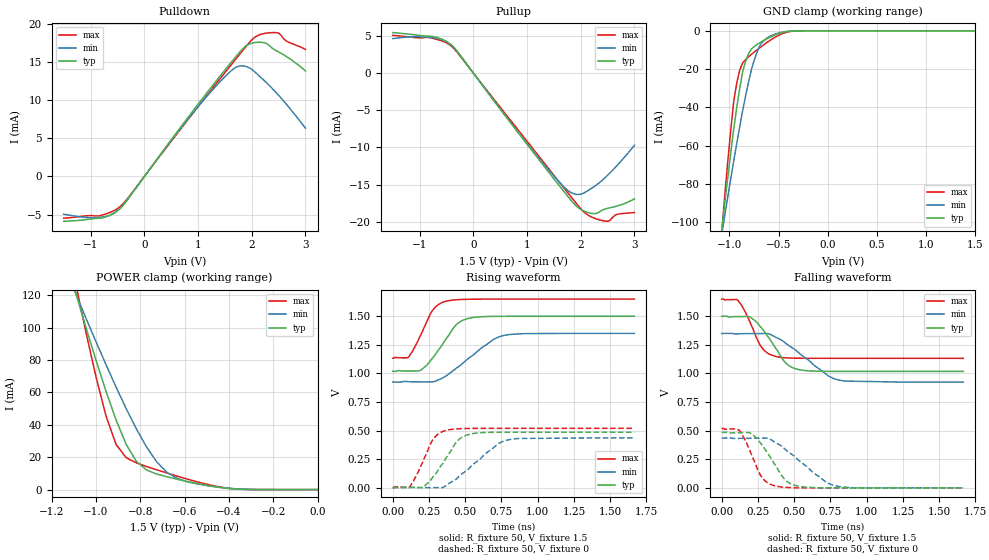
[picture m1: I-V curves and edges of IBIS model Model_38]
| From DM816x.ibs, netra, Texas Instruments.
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| Model based on original model for BSHTLTCSCDVGPBFZ
|   Sub model SLOWEST_4MA_10PER_1P5
[model]   Model_38
|[Description]  1.5V-3-STATE-X-SLOWEST, 4MA, +-10%
|[Input Load]
|[Output Drive] SLOWEST, 4MA
|Voltage   1.5V
|Mode   3-STATE
Model_type   3-state
Polarity   Non-Inverting
Enable   Active-Low
Cref =  15.0000pF
Rref =  100.0000M
Vref =  0V
Vmeas =  0.75
C_comp   1.5249p   1.4275p   1.6205p
[Model Spec]
[Temperature Range]   25   125   -40
[Voltage Range]   1.5   1.35   1.65
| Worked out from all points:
|   slope of the pulldown table from 0 to 0.225 V, typ, clamps not added: 103 ohm
|   slope of the pullup table from 0 to 0.225 V, typ, clamps not added: 103 ohm
|   GND clamp passes 1 mA (typ) near -0.47 V on its own axis
|   POWER clamp passes 1 mA (typ) near -0.42 V on its own axis
|   rising waveform, R_fixture 50, V_fixture 1.5: 20-80 % time 161ps typ, 258ps min, 118ps max; typ from 1.02 V to 1.5 V
|   rising waveform, R_fixture 50, V_fixture 0: 20-80 % time 154ps typ, 247ps min, 114ps max; typ from 0 V to 0.485 V
|   falling waveform, R_fixture 50, V_fixture 1.5: 20-80 % time 155ps typ, 264ps min, 113ps max; typ from 1.5 V to 1.02 V
|   falling waveform, R_fixture 50, V_fixture 0: 20-80 % time 150ps typ, 254ps min, 109ps max; typ from 0.485 V to 0 V
[POWER_clamp]
-1.5V     321.6mA    260.6mA    415.8mA
-1.091V   121.1mA    120.8mA    126.6mA
-1.076V   114.1mA    115.8mA    116.8mA
-1V       79.88mA    91.3mA     69.56mA
-954.5mV  60.58mA    77.05mA    45.34mA
-909.1mV  42.84mA    63.2mA     27.8mA
-818.2mV  17.47mA    37.6mA     16.51mA
-772.7mV  12.19mA    26.53mA    14.33mA
-681.8mV  7.985mA    10.89mA    10.33mA
-590.9mV  5.092mA    4.952mA    6.596mA
-363.6mV  298.9uA    465.6uA    298.1uA
0V        1.518nA    23.05nA    396.5pA
[Pulldown]
-1.5V     -5.88mA    -4.94mA    -5.47mA
-863.6mV  -5.487mA   -5.379mA   -5.186mA
-500mV    -4.486mA   -4.503mA   -4.211mA
-318.2mV  -3.077mA   -3.07mA    -2.94mA
1V        9.473mA    9.16mA     9.156mA
1.455V    13.57mA    12.77mA    13.23mA
1.727V    15.92mA    14.4mA     15.62mA
1.955V    17.38mA    14.26mA    17.57mA
2.273V    17.45mA    12.32mA    18.81mA
2.5V      16.34mA    10.65mA    18.81mA
2.636V    15.78mA    9.54mA     17.81mA
3V        13.85mA    6.33mA     16.67mA
[Pullup]
-1.5V     5.43mA     4.62mA     5.06mA
-772.7mV  4.923mA    4.757mA    4.681mA
-409.1mV  3.79mA     3.753mA    3.62mA
1.227V    -11.69mA   -11.51mA   -11.25mA
1.682V    -15.87mA   -15.27mA   -15.39mA
1.864V    -17.48mA   -16.22mA   -17.03mA
2V        -18.33mA   -16.3mA    -18.23mA
2.182V    -18.84mA   -15.6mA    -19.29mA
2.409V    -18.4mA    -14.37mA   -19.84mA
2.545V    -18.12mA   -13.43mA   -19.81mA
2.682V    -17.87mA   -12.4mA    -18.99mA
3V        -16.92mA   -9.72mA    -18.75mA
[GND_clamp]
-1.5V     -310mA     -250.5mA   -402.4mA
-1.076V   -103.5mA   -106.1mA   -105.2mA
-1.045V   -89.74mA   -96.32mA   -85.93mA
-954.5mV  -51.19mA   -67.85mA   -36.85mA
-924.2mV  -40.06mA   -58.84mA   -27.27mA
-863.6mV  -21.23mA   -41.55mA   -16.73mA
-833.3mV  -15.79mA   -33.74mA   -15.03mA
-772.7mV  -9.342mA   -19.74mA   -12.19mA
-712.1mV  -6.927mA   -10.35mA   -9.702mA
-621.2mV  -4.26mA    -3.894mA   -6.224mA
-409.1mV  -336.9uA   -288.9uA   -618.6uA
1.5V      1.518nA    2.298uA    269.6pA
[Ramp]
dV/dt_f   0.38584/0.22815933n   0.340824/0.36552773n   0.41424/0.17348723n
dV/dt_r 0.38899324/0.22248215n 0.35013688/0.34531566n 0.41519006/0.17156653n
R_load = 50
[Rising Waveform]
R_fixture = 50
V_fixture = 1.5
V_fixture_min = 1.35
V_fixture_max = 1.65
0s        1.018V     925mV      1.133V
108.7ps   1.02V      927.4mV    1.143V
197.4ps   1.032V     925.7mV    1.346V
274.1ps   1.133V     926.4mV    1.55V
371.3ps   1.308V     980.6mV    1.632V
425.4ps   1.408V     1.033V     1.643V
479.8ps   1.463V     1.085V     1.647V
686.8ps   1.499V     1.29V      1.65V
772.1ps   1.5V       1.334V     1.65V
1.667ns   1.5V       1.35V      1.65V
[Rising Waveform]
R_fixture = 50
V_fixture = 0
V_fixture_min = 0
V_fixture_max = 0
0s        0V         0V         0V
111.9ps   2.35mV     3.02mV     0V
207.2ps   0V         0V         224.2mV
285.7ps   107.1mV    0V         434.6mV
379.6ps   283.1mV    30.18mV    504.2mV
439.9ps   399.5mV    77.42mV    514mV
505.6ps   458.1mV    145mV      517.4mV
643.2ps   482.7mV    301.6mV    518.8mV
780.9ps   485.1mV    413.5mV    518.9mV
1.667ns   485.4mV    435.6mV    518.9mV
[Falling Waveform]
R_fixture = 50
V_fixture = 1.5
V_fixture_min = 1.35
V_fixture_max = 1.65
0s        1.499V     1.349V     1.649V
110.3ps   1.497V     1.346V     1.641V
200.1ps   1.49V      1.348V     1.435V
283.5ps   1.385V     1.349V     1.215V
383.2ps   1.2V       1.31V      1.145V
444.2ps   1.089V     1.261V     1.136V
510.9ps   1.04V      1.203V     1.133V
730.6ps   1.018V     983.2mV    1.132V
805.3ps   1.018V     942.8mV    1.132V
1.667ns   1.018V     924.1mV    1.132V
[Falling Waveform]
R_fixture = 50
V_fixture = 0
V_fixture_min = 0
V_fixture_max = 0
0s        484.8mV    434.8mV    518.3mV
123.4ps   482.7mV    432.6mV    499.7mV
200.5ps   476mV      434mV      308.1mV
272.8ps   383.1mV    434.4mV    100.8mV
362.4ps   212.1mV    402.6mV    18.6mV
433.1ps   76.69mV    342.7mV    5.178mV
494.5ps   25.82mV    283.5mV    0V
714.6ps   0V         55.28mV    0V
778.8ps   0V         19.48mV    0V
1.667ns   0V         0V         0V
